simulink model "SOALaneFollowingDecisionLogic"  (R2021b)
settings: Solver=FixedStepDiscrete  StartTime=0.0  StopTime=10.0  RelTol=1e-3

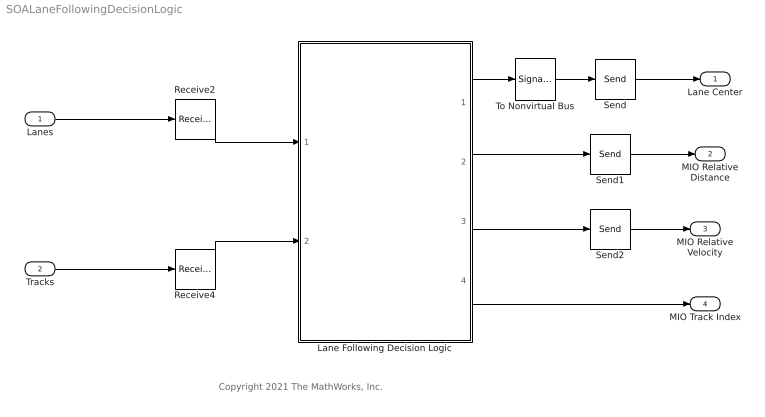
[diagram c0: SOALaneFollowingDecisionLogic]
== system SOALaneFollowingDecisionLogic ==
  note: Copyright 2021 The MathWorks, Inc.
  Lanes : Inport  OutputPortMessageModes=m  OutDataTypeStr=Bus: LaneSensor  PortDimensions=[1 1]
  Tracks : Inport  OutputPortMessageModes=m  Port=2  OutDataTypeStr=Bus: BusTrackerJPDA  PortDimensions=[1 1]
  Lane Following Decision Logic : ModelReference  ModelNameDialog=LaneFollowingDecisionLogic.slx  SimulationMode=Normal  ModelReferenceVersion=3.0
  Receive2 : Receive  InputPortMessageModes=m  UseInternalQueue=off  QueueOverwriting=on  QueueLength=1  QueueType=LIFO
  Receive4 : Receive  InputPortMessageModes=m  UseInternalQueue=off  QueueOverwriting=on  QueueLength=1  QueueType=LIFO
  Send : Send  OutputPortMessageModes=m
  Send1 : Send  OutputPortMessageModes=m
  Send2 : Send  OutputPortMessageModes=m
  To Nonvirtual Bus : SignalConversion  ConversionOutput=Nonvirtual bus  OverrideOpt=off
  Lane Center : Outport  InputPortMessageModes=m  OutDataTypeStr=Bus: BusLaneCenter
  MIO Relative Distance : Outport  InputPortMessageModes=m  Port=2
  MIO Relative Velocity : Outport  InputPortMessageModes=m  Port=3
  MIO Track Index : Outport  Port=4
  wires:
  Tracks/1 -> Receive4/1
  Lane Following Decision Logic/1 -> To Nonvirtual Bus/1
  Lanes/1 -> Receive2/1
  Receive2/1 -> Lane Following Decision Logic/1
  Lane Following Decision Logic/2 -> Send1/1
  Lane Following Decision Logic/3 -> Send2/1
  Receive4/1 -> Lane Following Decision Logic/2
  Send/1 -> Lane Center/1
  Send1/1 -> MIO Relative Distance/1
  Send2/1 -> MIO Relative Velocity/1
  To Nonvirtual Bus/1 -> Send/1
  Lane Following Decision Logic/4 -> MIO Track Index/1
